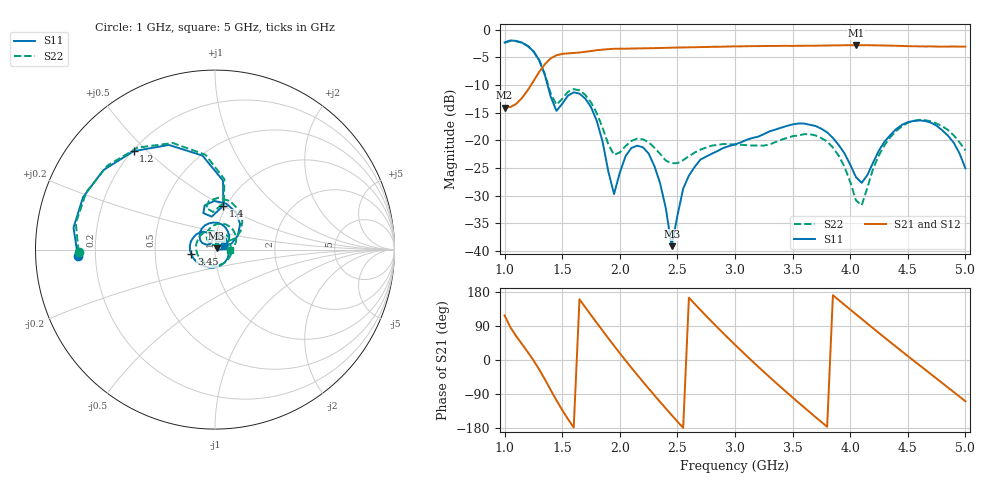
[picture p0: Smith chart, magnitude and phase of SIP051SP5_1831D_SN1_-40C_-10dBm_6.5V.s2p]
# GHz  S  dB  R  50
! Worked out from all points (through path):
!   81 points, 1 GHz to 5 GHz, reference 50 ohm
!   highest |S21| = -2.82 dB at 4.05 GHz (marker M1); lowest = -14.1 dB at 1 GHz (marker M2)
!   lowest |S11| = -39.1 dB at 2.45 GHz (marker M3), VSWR 1.02, Z = 50.9 + j0.665 ohm
!   |S11| at or under -10 dB: 1.373 GHz to end of sweep
!   |S22| runs from -31.7 to -2.1 dB; largest |S21 - S12| = 0.0016
!   S11 on the Smith chart (normalised r, x): 1 GHz: 0.13, -0.02; 1.2 GHz: 0.20, +0.45; 1.4 GHz: 0.97, +0.50; 3.45 GHz: 0.77, -0.04; 5 GHz: 1.11, +0.04
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1  -2.32 -177.4  -14.08 117.7  -14.08 117.6  -2.38 -179.1
1.2  -2.95 129.6  -10.97 21.4  -10.99 21.4  -2.94 127.1
1.4  -12.09 79.2  -5.20 -79.0  -5.20 -79.0  -11.52 79.2
1.55  -11.93 103.1  -4.29 -155.9  -4.29 -155.9  -11.24 97.0
1.7  -12.45 60.8  -4.01 139.3  -4.02 139.3  -11.78 58.8
1.85  -20.20 20.0  -3.62 77.7  -3.61 77.7  -17.71 29.1
1.95  -29.71 59.3  -3.47 37.6  -3.48 37.6  -22.63 45.7
2.05  -22.86 86.2  -3.45 -1.2  -3.44 -1.2  -21.03 62.0
2.2  -21.25 44.4  -3.38 -57.1  -3.40 -57.0  -19.81 42.8
2.35  -27.76 3.3  -3.32 -110.7  -3.31 -110.6  -22.45 28.5
2.45  -39.12 36.2  -3.27 -145.3  -3.27 -145.4  -24.14 32.5
2.55  -28.73 80.8  -3.23 -179.1  -3.21 -179.1  -23.58 39.3
2.75  -22.93 18.2  -3.14 116.2  -3.14 116.3  -21.30 22.0
3  -20.73 -65.7  -3.04 40.3  -3.03 40.3  -20.78 -30.2
3.2  -19.35 -116.7  -2.99 -17.2  -2.98 -17.2  -20.94 -92.8
3.45  -17.41 -169.1  -2.94 -85.6  -2.94 -85.6  -19.58 -179.5
3.7  -17.41 140.9  -2.91 -150.9  -2.90 -150.9  -19.12 110.7
3.85  -19.57 114.4  -2.86 171.0  -2.85 171.0  -21.30 78.1
4.05  -26.65 111.3  -2.82 120.8  -2.82 120.7  -30.84 76.0
4.35  -19.02 140.0  -2.91 46.6  -2.92 46.7  -19.39 113.5
4.65  -16.50 83.2  -3.05 -25.2  -3.06 -25.3  -16.38 56.3
5  -25.07 20.0  -3.07 -108.9  -3.08 -109.0  -21.82 -1.8
